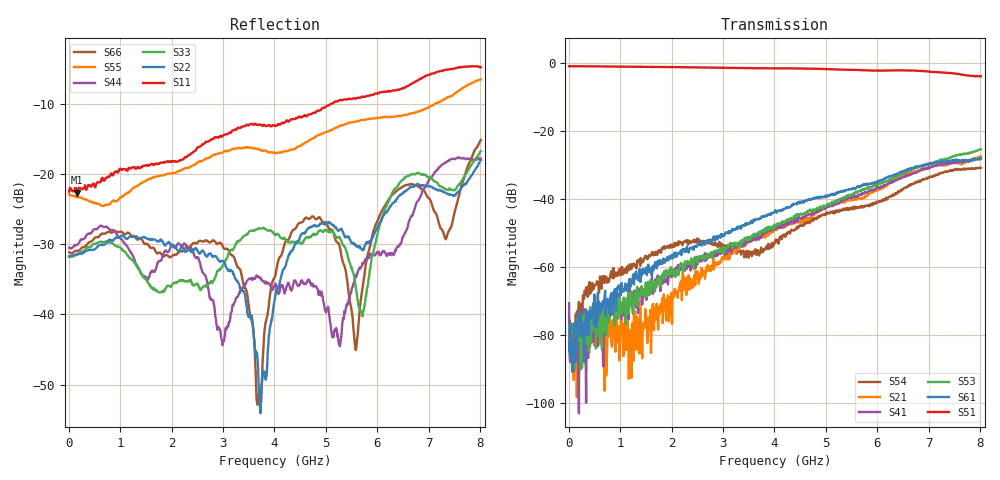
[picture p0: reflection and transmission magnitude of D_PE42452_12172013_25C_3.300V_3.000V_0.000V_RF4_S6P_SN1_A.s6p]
! Device ID: PE42422_06252012
! Dir: z:\David_A\42452\10_28_13_42452_omar_meas\25C\3p300000\RF4
! Serial: 1
! Insertion: A
! Temp: 25C
! VDD: 3.300
! Control_Hi: 3.000
! Control_Lo: 0.000
! Logic State: RF4
! Port 1: RFC
! Port 2: RF1
! Port 3: RF2
! Port 4: RF3
! Port 5: RF4
! Port 6: RF5
! ThroughPath:5-1
! V1 = 0.00
! V2 = 0.00
! V3 = 3.00
! V4 = 0.00
#  Hz  S  RI  R  50
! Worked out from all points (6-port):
!   801 points, 10 MHz to 8.01 GHz, reference 50 ohm
!   strongest paths, dB at 10 MHz, 2.01 GHz, 4.01 GHz, 6.01 GHz, 8.01 GHz:
!     S51: -0.8, -1.1, -1.4, -2.1, -3.7
!     S61: -82.1, -56.3, -43.8, -34.7, -28.1
!     S53: -77.3, -62.2, -48.1, -35.4, -25.3
!     S41: -70.6, -61.7, -48.6, -36.6, -28.0
!     S21: -78.3, -76.7, -48.8, -37.1, -27.3
!     S54: -81.8, -53.8, -52.4, -40.9, -30.8
!   lowest |S11| = -22.7 dB at 170 MHz (marker M1), VSWR 1.16, Z = 57.7 - j1.89 ohm
!   |S11| at or under -10 dB: start of sweep to 5.112 GHz
